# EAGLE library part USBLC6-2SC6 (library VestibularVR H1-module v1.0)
TVS DIODE 5.25VWM 17VC SOT23-6
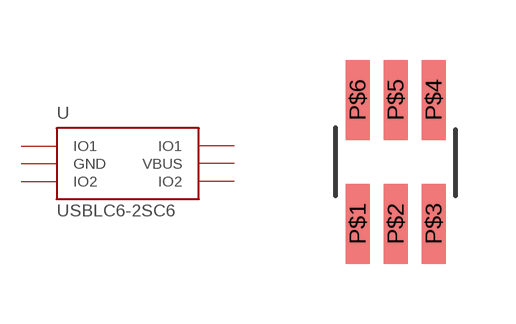
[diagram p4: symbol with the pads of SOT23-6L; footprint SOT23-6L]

Designator prefix -

## USBLC6-2SC6  [SOT23-6L]
P$1  IO1
P$2  GND
P$3  IO2
P$4  IO2
P$5  VBUS
P$6  IO1

## Footprint SOT23-6L (pad centres in mm)
smd 0.6 x 2: P$1 -0.95,-1.55; P$2 0,-1.55; P$3 0.95,-1.55; P$4 0.95,1.55; P$5 0,1.55; P$6 -0.95,1.55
